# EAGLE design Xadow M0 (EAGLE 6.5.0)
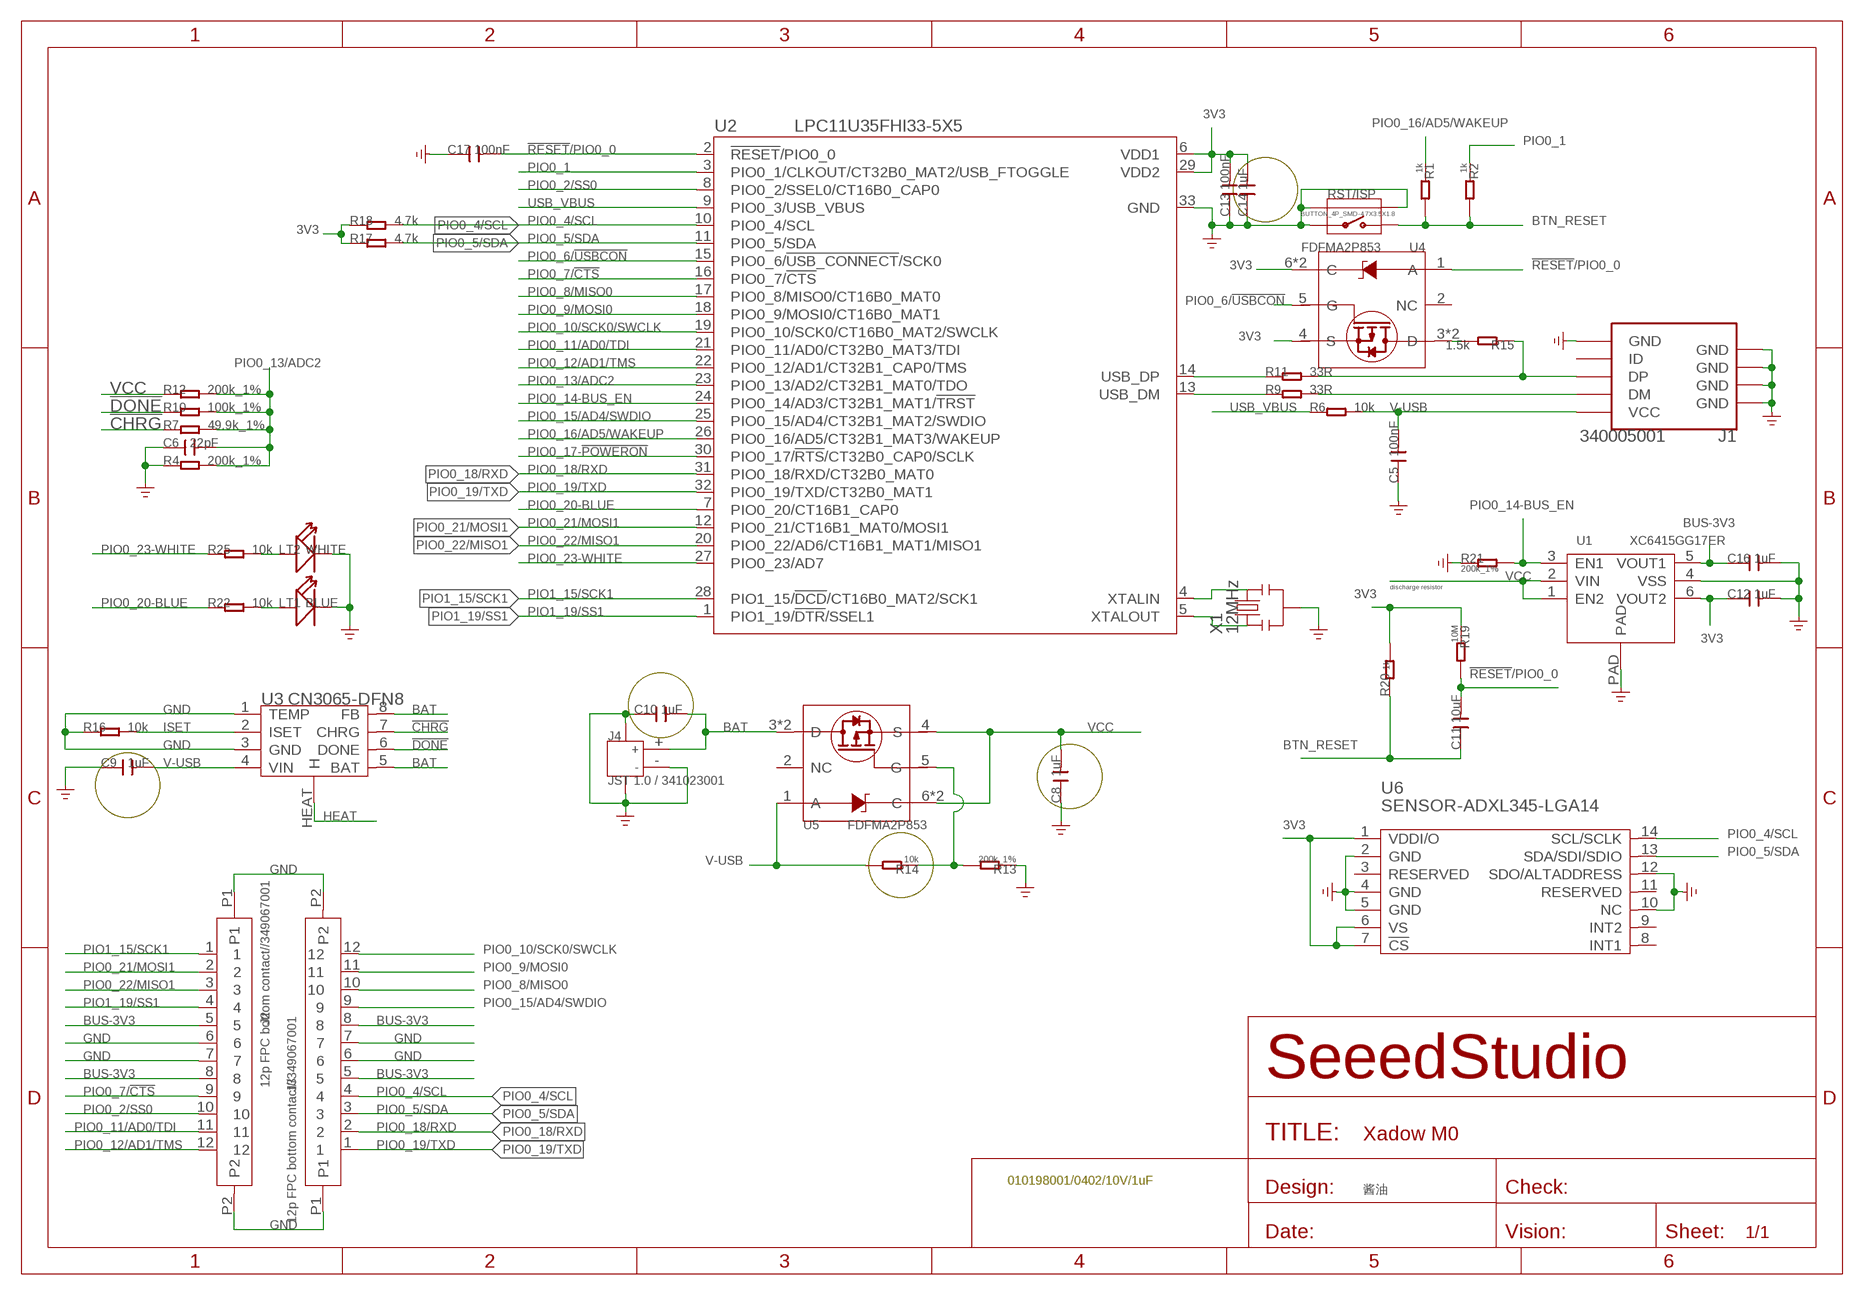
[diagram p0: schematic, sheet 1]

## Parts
C5  100nF  C-0402  [C0402]
C6  22pF  C-0402  [C0402]
C8  1uF  C-0402  [C0402]
C9  1uF  C-0402  [C0402]
C10  1uF  C-0402  [C0402]
C11  10uF  C-0402  [C0402]
C12  1uF  C-0402  [C0402]
C13  100nF  C-0402  [C0402]
C14  1uF  C-0402  [C0402]
C16  1uF  C-0402  [C0402]
C17  100nF  C-0402  [C0402]
J1  340005001  USB-MINIUSB-5P-MICRO  [MICRO-USB]
J2  12p FPC bottom contact//349067001  FPC052002-12LT-FH12-12S-0.5SH  [12P-0.5-NEW]
J3  12p FPC bottom contact//349067001  FPC052002-12LT-FH12-12S-0.5SH  [12P-0.5-NEW]
J4  JST 1.0 / 341023001  JACK-JST-2P-SMD-PW'1.0'  [JST-SMD-2P-1.0-90D]
LT1  BLUE  LED'0402'  [LED-0402]
LT2  WHITE  LED'0402'  [LED-0402]
R1  1k  R-0402  [R0402]
R2  1k  R-0402  [R0402]
R4  200k_1%  R-0402  [R0402]
R6  10k  R-0402  [R0402]
R7  49.9k_1%  R-0402  [R0402]
R9  33R  R-0402  [R0402]
R10  100k_1%  R-0402  [R0402]
R11  33R  R-0402  [R0402]
R12  200k_1%  R-0402  [R0402]
R13  200k_1%  R-0402  [R0402]
R14  10k  R-0402  [R0402]
R15  1.5k  R-0402  [R0402]
R16  10k  R-0402  [R0402]
R17  4.7k  R-0402  [R0402]
R18  4.7k  R-0402  [R0402]
R19  10M  R-0402  [R0402]
R20  1k  R-0402  [R0402]
R21  200k_1%  R-0402  [R0402]
R22  10k  R-0402  [R0402]
R25  10k  R-0402  [R0402]
RST/ISP  BUTTON_4P_SMD-4.7X3.5X1.8  [4P-SMD-4.7X3.5X1.8]
U1  XC6415GG17ER  XC6415  [USP-6C]
U2  LPC11U35FHI33-5X5  [HVQFN33]
U3  CN3065-DFN8  [DFN8]
U4  FDFMA2P853  [6P-SMD-W/-HEAT]
U5  FDFMA2P853  [6P-SMD-W/-HEAT]
U6  SENSOR-ADXL345-LGA14  [LGA14]
X1  12MHz  CRYSTAL-RESONATOR'SMD'  [3P-SMD-3.6X1.3]

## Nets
3V3: C12.1 C13.2 C14.2 R17.1 R18.1 R19.1 R20.2 U1.6(VOUT2) U2.6(VDD1) U2.29(VDD2) U4.4(S) U4.6(C) U4.P1(C) U6.1(VDDI/O) U6.6(VS) U6.7(!CS)
!CHRG: R7.1 U3.7(CHRG)
!DONE: R10.1 U3.6(DONE)
!RESET!/PIO0_0: C11.2 C17.2 R19.2 U2.2(!RESET!/PIO0_0) U4.1(A)
BAT: C10.2 J4.+ U3.5(BAT) U3.8(FB) U5.3(D) U5.P2(D)
BTN_RESET: C11.1 R1.2 R2.2 R20.1 RST/ISP.2
BUS-3V3: C16.1 J2.5 J2.8 J3.5 J3.8 U1.5(VOUT1)
GND: C5.1 C6.1 C8.1 C9.1 C10.1 C12.2 C13.1 C14.1 C16.2 C17.1 J1.5(GND) J1.S1(GND) J1.S2(GND) J1.S3(GND) J1.S4(GND) J1.S5(GND) J1.S6(GND) J2.6 J2.7 J2.P1 J2.P2 J3.6 J3.7 J3.P1 J3.P2 J4.3 J4.4 J4.- LT1.- LT2.- R4.1 R13.1 R16.1 R21.1 RST/ISP.1 RST/ISP.S1 RST/ISP.S2 U1.4(VSS) U1.PAD U2.33(GND) U3.1(TEMP) U3.3(GND) U6.2(GND) U6.4(GND) U6.5(GND) U6.10(NC) U6.12(SDO/ALTADDRESS) X1.2
HEAT: U3.HEAT(H)
ISET: R16.2 U3.2(ISET)
N$1: R11.1 U2.14(USB_DP)
N$2: R9.1 U2.13(USB_DM)
N$3: J1.2(DM) R9.2
N$4: J1.3(DP) R11.2 R15.1
N$5: LT2.+ R25.2
N$6: U2.4(XTALIN) X1.3
N$7: U2.5(XTALOUT) X1.1
N$8: R13.2 R14.1 U5.5(G)
N$9: LT1.+ R22.2
N$11: R15.2 U4.3(D) U4.P2(D)
PIO0_1: R2.1 U2.3(PIO0_1/CLKOUT/CT32B0_MAT2/USB_FTOGGLE)
PIO0_2/SS0: J2.10 U2.8(PIO0_2/SSEL0/CT16B0_CAP0)
PIO0_4/SCL: J3.4 R18.2 U2.10(PIO0_4/SCL) U6.14(SCL/SCLK)
PIO0_5/SDA: J3.3 R17.2 U2.11(PIO0_5/SDA) U6.13(SDA/SDI/SDIO)
PIO0_6/!USBCON: U2.15(PIO0_6/!USB_CONNECT!/SCK0) U4.5(G)
PIO0_7/!CTS: J2.9 U2.16(PIO0_7/!CTS!)
PIO0_8/MISO0: J3.10 U2.17(PIO0_8/MISO0/CT16B0_MAT0)
PIO0_9/MOSI0: J3.11 U2.18(PIO0_9/MOSI0/CT16B0_MAT1)
PIO0_10/SCK0/SWCLK: J3.12 U2.19(PIO0_10/SCK0/CT16B0_MAT2/SWCLK)
PIO0_11/AD0/TDI: J2.11 U2.21(PIO0_11/AD0/CT32B0_MAT3/TDI)
PIO0_12/AD1/TMS: J2.12 U2.22(PIO0_12/AD1/CT32B1_CAP0/TMS)
PIO0_13/ADC2: C6.2 R4.2 R7.2 R10.2 R12.2 U2.23(PIO0_13/AD2/CT32B1_MAT0/TDO)
PIO0_14-BUS_EN: R21.2 U1.3(EN1) U2.24(PIO0_14/AD3/CT32B1_MAT1/!TRST!)
PIO0_15/AD4/SWDIO: J3.9 U2.25(PIO0_15/AD4/CT32B1_MAT2/SWDIO)
PIO0_16/AD5/WAKEUP: R1.1 U2.26(PIO0_16/AD5/CT32B1_MAT3/WAKEUP)
PIO0_17-!POWERON: U2.30(PIO0_17/!RTS!/CT32B0_CAP0/SCLK)
PIO0_18/RXD: J3.2 U2.31(PIO0_18/RXD/CT32B0_MAT0)
PIO0_19/TXD: J3.1 U2.32(PIO0_19/TXD/CT32B0_MAT1)
PIO0_20-BLUE: R22.1 U2.7(PIO0_20/CT16B1_CAP0)
PIO0_21/MOSI1: J2.2 U2.12(PIO0_21/CT16B1_MAT0/MOSI1)
PIO0_22/MISO1: J2.3 U2.20(PIO0_22/AD6/CT16B1_MAT1/MISO1)
PIO0_23-WHITE: R25.1 U2.27(PIO0_23/AD7)
PIO1_15/SCK1: J2.1 U2.28(PIO1_15/!DCD!/CT16B0_MAT2/SCK1)
PIO1_19/SS1: J2.4 U2.1(PIO1_19/!DTR!/SSEL1)
USB_VBUS: R6.1 U2.9(PIO0_3/USB_VBUS)
V-USB: C5.2 C9.2 J1.1(VCC) R6.2 R14.2 U3.4(VIN) U5.1(A)
VCC: C8.2 R12.1 U1.1(EN2) U1.2(VIN) U5.4(S) U5.6(C) U5.P1(C)
Unconnected: J1.4(ID) U4.2(NC) U5.2(NC) U6.3(RESERVED) U6.8(INT1) U6.9(INT2) U6.11(RESERVED)

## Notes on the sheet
- discharge resistor
- 010198001/0402/10V/1uF
- 酱油

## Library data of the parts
C5 C6 C8-C14 C16 C17 = Discrete:C*: Ceramic Capacitors
J1 = Connector :USB-MINIUSB-5P
J2 J3 = template:FPC052002-12LT
J4 = Connector :JACK-JST-2P-SMD-PW
LT1 LT2 = Discrete:LED*
R1 R2 R4 R6 R7 R9-R22 R25 = Discrete:R*
RST/ISP = For_Test_Albert:BUTTON_4P_SMD: TS-1188E http://www.best-dz.com/?thread-374-2.html
U1 = template :XC6415: Dual LDO Regulator with ON/OFF Switch
U2 = For_Test_Albert:LPC11U35FHI33
U3 = IC:CN3065: USB-Compatible Lithiumt-Ion Battery Charger with Thermal Regulation http://www.consonance-elec.com/pdf/%E6%8A%80%E6%9C%AF%E8%AF%B4%E6%98%8E%E4%B9%A6/DSC-CN3065.pdf
U4 = template:FDFMA2P853: Integrated P-Channel Power Trench MOSFET and Schottky Diode
U5 = template :FDFMA2P853: Integrated P-Channel Power Trench MOSFET and Schottky Diode
U6 = Discrete:SENSOR-ADXL345: 3-Axis,+/-2g / +/-4g / +/-8g / +/-16g Digital Accelerometer http://www.analog.com/static/imported-files/data_sheets/ADXL345.pdf
X1 = Discrete:CRYSTAL-RESONATOR: Resonator Small SMD resonator. This is the itty bitty 10/20MHz resonators with built in caps. CSTCE10M0G55 and CSTCE20M0V53. Footprint has been reviewed closely but hasn't been tested yet.

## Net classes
0 default: width 0.102 mm, drill 0.203 mm, clearance 0.102 mm

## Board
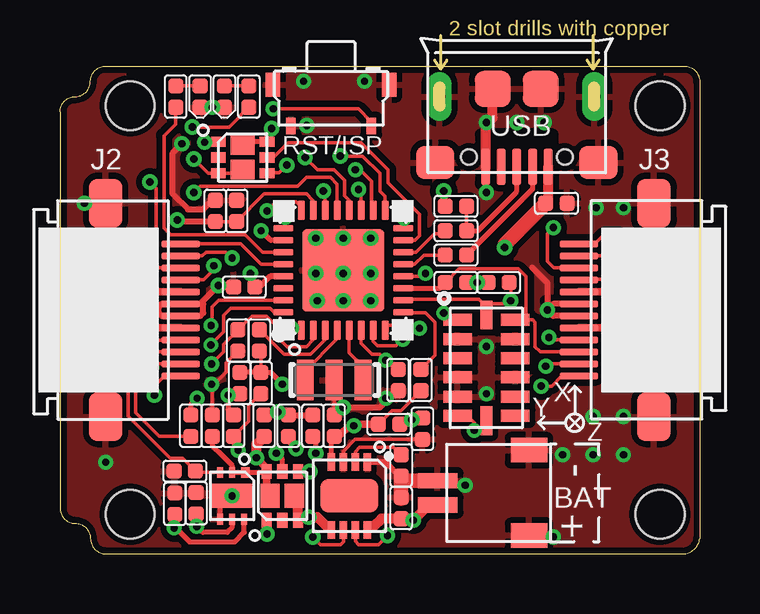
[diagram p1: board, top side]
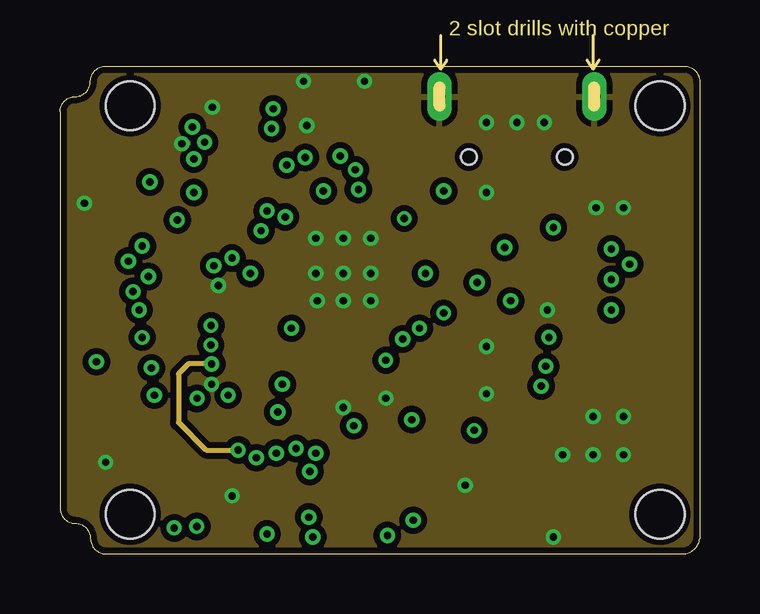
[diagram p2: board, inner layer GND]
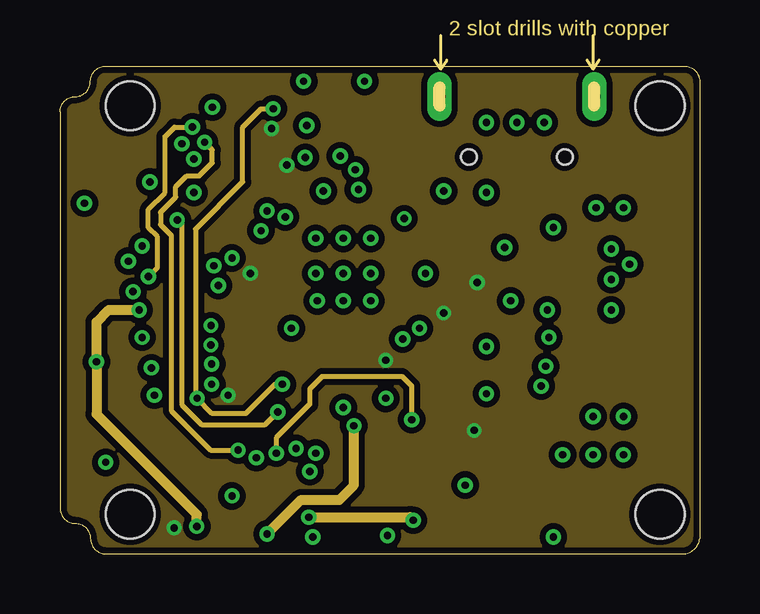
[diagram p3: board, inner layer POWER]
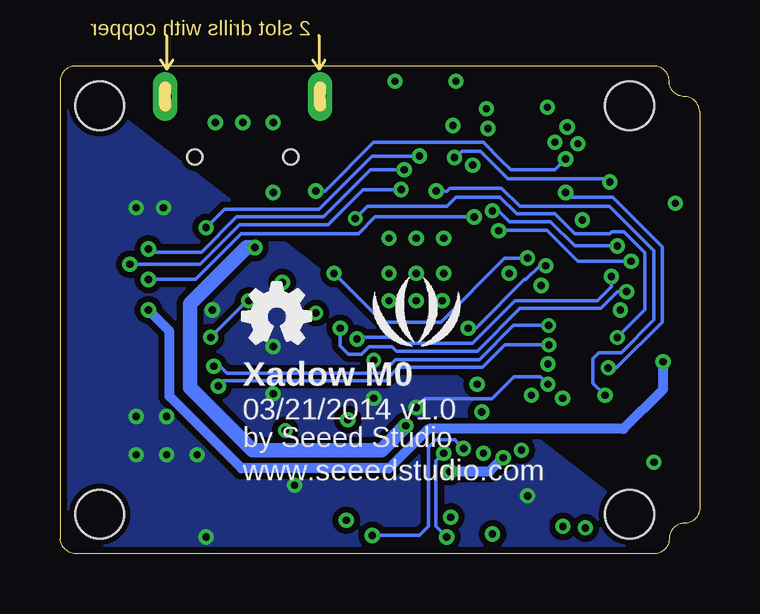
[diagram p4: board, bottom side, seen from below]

Size 26.67 x 20.32 mm. Coordinates in mm from the lower left corner, seen from the top.
Outline: 25.91,0 arc90 26.67,0.64
Outline: 26.04,20.32 arc-90 26.67,19.69
Outline: 1.27,19.69 arc-90 1.91,20.32
Outline: 0,1.91 arc90 0.64,1.27
Outline: 0,18.42 arc-90 0.64,19.05
Outline: 0.64,19.05 arc90 1.27,19.69
Outline: 0.64,1.27 arc-90 1.27,0.64
Outline: 1.27,0.64 arc90 1.91,0
Outline: 25.91,0 arc90 26.67,0.64
Outline: 26.04,20.32 arc-90 26.67,19.69
Outline: 26.67,19.69 26.67,0.64
Outline: 1.27,19.69 arc-90 1.91,20.32
Outline: 0,18.42 0,1.91
Outline: 0,1.91 arc90 0.64,1.27
Outline: 0,18.42 arc-90 0.64,19.05
Outline: 0.64,19.05 arc90 1.27,19.69
Outline: 0.64,1.27 arc-90 1.27,0.64
Outline: 1.27,0.64 arc90 1.91,0
Outline: 1.91,0 25.91,0
Outline: 1.91,20.32 26.04,20.32
Copper layers (1*2*15*16): Top 0.035mm / dielectric 0.2mm / GND 0.0175mm / dielectric 0.3mm / POWER 0.0175mm / dielectric 0.2mm / Bottom 0.035mm
Design rules "default *": minimum track width 6mil, minimum drill 12mil, track to track 6mil, track to pad 6mil, pad to pad 6mil, via to via 6mil, smd to smd 0mil, copper to edge 6mil, drill to drill 10mil, minimum pad ring 6mil, minimum via ring 6mil, stop-mask expansion 2mil, vias tented up to drill 25mil, thermal gap 10mil
Holes 2.03 mm at 2.92,1.65 25.02,18.67 25.02,1.65 2.92,18.67
tRestrict: area 20.3,9.8 to 21.5,10.5; area 3.9,9.8 to 5.1,10.5; area 9.1,6.6 to 16.3,13.8; 1 lines
bRestrict: 1 lines

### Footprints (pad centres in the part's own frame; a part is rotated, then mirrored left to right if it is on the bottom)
C0402 = smd 0.635 x 0.635: 1 -0.445,0; 2 0.445,0
MICRO-USB = smd 0.381 x 1.524: 1 -1.3,-0.25; 2 -0.65,-0.25; 3 0,-0.25; 4 0.65,-0.25; 5 1.3,-0.25 | smd 1.6 x 1.397: S1 -3.4,-0.427; S6 3.4,-0.427 | drill 0.508 pad 1.016 long: S2 -3.226,-3.175; S5 3.226,-3.175 | smd 1.5 x 1.5: S3 -1,-3.5; S4 1,-3.5 | hole 0.635: -2,-0.65; 2,-0.65
12P-0.5-NEW = smd 0.3 x 1.6: 1 -2.75,3.127; 2 -2.25,3.127; 3 -1.75,3.127; 4 -1.25,3.127; 5 -0.75,3.127; 6 -0.25,3.127; 7 0.25,3.127; 8 0.75,3.127; 9 1.25,3.127; 10 1.75,3.127; 11 2.25,3.127; 12 2.75,3.127 | smd 2.032 x 1.397: P1 -4.445,0; P2 4.445,0
JST-SMD-2P-1.0-90D = smd 1.524 x 1.016: 3 -3.429,1.778; 4 -3.429,-1.778 | smd 1.651 x 0.635: + 0.381,0.508; - 0.381,-0.508
LED-0402 = smd 0.635 x 0.635: + -0.445,0; - 0.445,0
R0402 = smd 0.635 x 0.635: 1 -0.445,0; 2 0.445,0
4P-SMD-4.7X3.5X1.8 = smd 0.4 x 0.7: 1 -1.675,-1.227; 2 1.675,-1.227 | smd 0.6 x 1: S1 -2.425,0.5; S2 2.425,0.5
USP-6C = smd 0.45 x 0.35: 1 -0.975,0.55 | smd 0.45 x 0.25: 2 -0.975,0; 3 -0.975,-0.5; 4 0.975,-0.5; 5 0.975,0; 6 0.975,0.5 | smd 1 x 1.8: PAD 0,0
HVQFN33 = smd 0.813 x 0.279: 1 -2.5,1.75; 2 -2.5,1.25; 3 -2.5,0.75; 4 -2.5,0.25; 5 -2.5,-0.25; 6 -2.5,-0.75; 7 -2.5,-1.25; 8 -2.5,-1.75; 17 2.5,-1.75; 18 2.5,-1.25; 19 2.5,-0.75; 20 2.5,-0.25; 21 2.5,0.25; 22 2.5,0.75; 23 2.5,1.25; 24 2.5,1.75 | smd 0.279 x 0.813: 9 -1.75,-2.5; 10 -1.25,-2.5; 11 -0.75,-2.5; 12 -0.25,-2.5; 13 0.25,-2.5; 14 0.75,-2.5; 15 1.25,-2.5; 16 1.75,-2.5; 25 1.75,2.5; 26 1.25,2.5; 27 0.75,2.5; 28 0.25,2.5; 29 -0.25,2.5; 30 -0.75,2.5; 31 -1.25,2.5; 32 -1.75,2.5 | smd 3.429 x 3.429: 33 0,0
DFN8 = smd 0.3 x 0.727: 1 -0.75,-1.413; 2 -0.25,-1.413; 3 0.25,-1.413; 4 0.75,-1.413; 5 0.75,1.413; 6 0.25,1.413; 7 -0.25,1.413; 8 -0.75,1.413 | smd 2.413 x 1.397: HEAT 0,0
6P-SMD-W/-HEAT = smd 0.42 x 0.62: 1 -0.65,-1.015; 2 0,-1.015; 3 0.65,-1.015; 4 0.65,1.015; 5 0,1.015; 6 -0.65,1.015 | smd 0.8 x 1: P1 -0.508,0; P2 0.5,0
LGA14 = smd 1.2 x 0.5: 1 -1.2,2; 2 -1.2,1.2; 3 -1.2,0.4; 4 -1.2,-0.4; 5 -1.2,-1.2; 6 -1.2,-2; 8 1.2,-2; 9 1.2,-1.2; 10 1.2,-0.4; 11 1.2,0.4; 12 1.2,1.2; 13 1.2,2 | smd 0.5 x 1.2: 7 0,-2.2; 14 0,2.2
3P-SMD-3.6X1.3 = smd 0.7 x 1.7: 1 -1.2,0; 2 0,0; 3 1.2,0

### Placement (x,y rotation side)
C5  20.7,14.61 180 top
C6  7.37,14.29 270 top
C8  6.35,5.34 270 top
C9  11.43,5.34 270 top
C10  14.22,1.91 270 top
C11  8.38,7.11 270 top
C12  4.79,2.09 90 top
C13  7.68,11.12 0 top
C14  14.1,7.24 90 top
C16  5.68,2.11 90 top
C17  7.42,8.89 90 top
J1  19.05,15.88 180 top
J2  1.91,10.16 270 top
J3  24.76,10.16 90 top
J4  16.13,2.54 180 top
LT1  6.86,19.05 270 top
LT2  5.84,19.05 270 top
R1  5.46,5.34 90 top
R2  8.31,8.89 270 top
R4  6.48,14.29 270 top
R6  15.05,7.24 270 top
R7  9.53,5.34 90 top
R9  16.51,12.45 0 top
R10  10.54,5.34 90 top
R11  16.51,13.46 0 top
R12  8.51,5.34 90 top
R13  15.11,5.21 90 top
R14  13.72,5.4 180 top
R15  16.51,14.48 180 top
R16  14.22,3.69 90 top
R17  16.51,11.31 180 top
R18  18.29,11.31 0 top
R19  7.24,5.34 270 top
R20  7.49,7.11 270 top
R21  5.21,3.44 0 top
R22  7.87,19.05 90 top
R25  4.83,19.05 90 top
RST/ISP  11.3,19.05 0 top
U1  7.18,2.42 270 top
U2  11.81,11.81 90 top
U3  12.06,2.42 180 top
U4  7.62,16.51 270 top
U5  9.27,2.42 0 top
U6  17.78,7.75 0 top
U$13  [OSHW_FILLX100_NOTEXT]  19.05,8.77 0 bottom
U$14  [SILK_SCREEN_150X124]  11.81,9.78 0 bottom
X1  11.43,7.24 180 top

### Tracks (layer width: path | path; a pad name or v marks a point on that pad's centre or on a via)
3V3  (via drill 0.3 pad 0.61, 0.3 pad 0.64)
  Top 0.152: U4.4 8.75,15.86 8.76,15.88 9.14,15.88 v9.46,16.2 | U2.6 12.56,8.78 13.02,8.32 13.34,8.32 v13.59,8.07 13.97,7.69 C14.2 | U6.7 17.78,5.21 17.72,5.15 v17.27,5.15 17.27,5.46 17.02,5.72 16.61,5.72 U6.6 | R18.1 v17.4,11.31 | 7.37,5.91 R19.1 | U6.1 16.29,9.75 v16,10.04
  Top 0.203: C12.1 4.79,1.12 5.41,0.5 7.29,0.5 7.68,0.89 U1.6 | v8.83,17.72 8.63,17.53 U4.6 7.76,17.16 U4.P1 | R20.2 7.07,6.67 v7.01,6.61 7.01,6.01 R19.1
  Top 0.254: v7.94,11.69 7.94,11.31 C13.2 8.19,11.05 8.26,11.05 8.77,11.56 U2.29
  Top 0.305: C12.1 4.79,1.11 v4.76,1.08
  Top 0.406: R17.1 v17.4,11.31
  pour POWER (isolate 0.254): 27.3,20.32 -3.17,20.32 -3.17,-0.63 27.3,-0.63
!CHRG  (via drill 0.3 pad 0.64)
  Top 0.152: U3.7 12.31,0.51 12.45,0.38 13.27,0.38 v13.65,0.76
  Top 0.203: 9.53,4.83 R7.1 9.53,4.7 v9.84,4.38
  Bottom 0.152: v13.65,0.76 11.68,0.76 11.3,1.15 11.3,4.44 11,4.74 10.2,4.74 10.08,4.62 v9.84,4.38
!DONE  (via drill 0.3 pad 0.64)
  Top 0.152: U3.6 11.81,0.51 11.69,0.38 10.86,0.38 v10.54,0.7
  Top 0.203: v10.67,4.19 10.67,4.76 R10.1
  Bottom 0.152: v10.67,4.19 10.98,3.88 10.98,1.15 v10.54,0.7
!RESET!/PIO0_0  (via drill 0.3 pad 0.64)
  Top 0.152: U2.2 10.56,8.91 10.29,8.64 9.47,8.64 9.02,9.1 9.02,9.5 8.61,9.91 8,9.91 7.6,9.5 7.58,9.5 C17.2 6.83,8.74 6.83,8.42 v6.33,7.91 | U4.1 6.05,17.16 v6.03,17.15 | C11.2 7.87,6.16 7.87,5.53 R19.2 7.24,4.51 v7.43,4.32
  GND 0.203: v7.43,4.32 6.1,4.32 4.94,5.47 4.94,7.5 5.36,7.91 v6.33,7.91
  POWER 0.203: v7.43,4.32 6.28,4.32 4.64,5.97 4.64,13.27 4.19,13.72 4.19,14.23 4.83,14.86 4.83,15.29 5.28,15.75 5.81,15.75 6.35,16.29 6.35,16.83 v6.03,17.15
BAT  (via drill 0.3 pad 0.64)
  Top 0.254: 12.95,1.15 12.95,1.14 U3.8
  Top 0.305: U3.8 | 11.18,1.08 11.23,1.08 U3.5
  Top 0.406: U5.3 9.92,1.53 | 9.92,1.53 9.92,2.27 U5.P2 | J4.+ 15.37,2.03 v14.73,1.4 14.29,1.4 C10.2 13.4,1.46 13.08,1.15 12.95,1.15 | 9.92,1.53 v10.38,1.53 10.73,1.53 11.18,1.08
  POWER 0.406: v10.38,1.53 14.6,1.53 v14.73,1.4
BTN_RESET  (via drill 0.3 pad 0.64)
  Top 0.152: 12.95,17.8 RST/ISP.2 12.98,18.01 12.45,18.54 v8.89,18.54 | C11.1 8.38,8.37 R2.2
  Top 0.203: R20.1 C11.1 8.78,7.56 v9.27,7.06 | R1.2 5.46,6.23 v5.71,6.48
  POWER 0.203: v8.89,18.54 8.38,18.54 7.62,17.78 7.62,15.5 5.65,13.53 5.65,6.54 v5.71,6.48 6.35,5.84 7.75,5.84 8.97,7.06 v9.27,7.06
BUS-3V3  (via drill 0.3 pad 0.64)
  Top 0.203: U1.5 7.18,1.09 6.98,0.9 5.95,0.9 v5.7,1.15 5.7,1.6 | 5.7,1.6 5.7,1.64 C16.1 | 5.7,1.6 5.65,1.65 | 21.65,10.92 J3.8
  Top 0.254: 5.02,9.4 J2.8
  Top 0.305: J2.8 4.04,9.41 4.04,9.42 v3.3,10.16 4.04,10.91 J2.5 | J3.5 22.64,9.41 22.99,9.76 v22.99,10.16 22.99,10.54 22.62,10.91 J3.8
  POWER 0.406: v3.3,10.16 2.03,10.16 1.52,9.65 v1.52,8 1.52,5.82 5.7,1.64 v5.7,1.15
  Bottom 0.406: v22.99,10.16 22.1,9.27 22.1,6.56 19.1,3.56 12.95,3.56 11.3,5.21 3.17,5.21 1.52,6.86 v1.52,8
GND  (via drill 0.3 pad 0.64)
  Top 0.152: LT2.- v6.35,18.61 LT1.- | U3.3 11.81,4.27 12.31,4.76 R13.1 | C17.1 6.92,7.95 6.92,7.56 6.43,7.06 v6.33,7.06 6.35,7.04 C8.1 | X1.2 11.43,6.1 v11.81,6.1
  Top 0.203: U1.4 6.68,2.3 6.79,2.42 U1.PAD
  Top 0.254: 5.84,10.41 J2.6 4.24,10.42 4.09,10.26 4.09,10.07 4.24,9.91 J2.7 5.85,9.91 5.97,10.04 5.97,10.42 | 5.84,10.41 5.97,10.54 | C13.1 6.54,11.11 | U3.1 13.57,3.83 14.22,3.18 14.16,3.18 R16.1 | 5.97,10.42 5.97,10.54 | 5.97,10.54 6.54,11.11 | 6.54,11.11 v6.6,11.18 | 5.84,10.41 5.96,10.41 5.97,10.42 | 21.47,10.41 J3.7 20.57,10.41 v20.32,10.16 | 21.72,9.91 21.71,9.91 J3.6 20.57,9.91 v20.32,10.16 | v13.59,6.48 13.59,6.35 13.34,6.1 v11.81,6.1 11.56,6.1 | 19.68,11.94 20.32,11.31 v20.32,10.16 | R4.1 6.35,14.73 5.97,14.35 5.33,14.35 4.7,14.99 4.7,16.7 v5.08,17.08
  Top 0.305: J2.P1 v1.02,14.61
  Top 0.406: 17.75,17.88 18.03,18.16 18.03,19.36 J1.S4 | 11.56,6.1 11.56,5.91 C9.1 | J1.5 17.75,18.01 17.78,18.04
  Top 0.61: J4.- 14.22,3.05 | 14.22,3.05 14.22,3.18 R16.1 | 14.22,3.05 14.22,2.29 | U2.33 11.81,11.88
  Bottom 0.152: v6.33,7.06 6.63,7.37 7.75,7.37 8.66,6.45 11.46,6.45 v11.81,6.1
  other vias: 23.49,5.72 10.73,10.54 11.81,10.54 12.95,10.54 10.29,17.85 10.16,19.69 20.95,4.13 16.89,2.86 20.57,0.7 17.78,17.97 19.05,17.97 20.19,17.97 10.67,13.15 11.81,13.15 12.95,13.15 11.81,11.69 10.67,11.69 12.95,11.69 7.18,2.42 1.91,3.81 17.78,8.64 17.78,15.05 22.35,14.42 12.7,19.69 17.78,6.67 23.49,14.42 22.22,5.72 22.22,4.13 23.49,4.13
  pour GND (isolate 0.254): 27.3,20.32 -2.54,20.32 -2.54,-0.63 27.3,-0.63
  pour Bottom (isolate 0.254, rank 4): 27.3,20.7 27.3,-0.63 -0.25,-0.63
  pour Top (isolate 0.254, rank 4): -0.25,20.7 27.3,20.7 27.3,-0.63 -0.25,-0.63
ISET
  Top 0.152: U3.2 12.31,4.26 12.49,4.44 13.91,4.44 R16.2 | R16.2 14.29,4.13 | 14.1,4.26 R16.2
N$1
  Top 0.152: U2.14 14.85,12.56 15.62,13.34 15.94,13.34 R11.1
N$2
  Top 0.152: U2.13 14.79,12.06 15.18,12.45 R9.1
N$3
  Top 0.203: J1.2 19.7,15.19 18.61,14.1 17.53,13.02 R9.2
N$4
  Top 0.152: R15.1 R11.2
  Top 0.203: R11.2 17.42,13.46 19.05,15.09 J1.3
N$5
  Top 0.152: R25.2 LT2.+
N$6
  Top 0.152: U2.4 11.56,8.96 10.23,7.63 X1.3
N$7
  Top 0.152: U2.5 12.06,8.39 12.64,7.81 12.64,7.25 X1.1
N$8  (via drill 0.3 pad 0.64)
  Top 0.203: U5.5 9.27,3.94 v9.02,4.19
  Top 0.254: R14.1 14.48,5.4 v14.67,5.59 14.73,5.65 R13.2
  POWER 0.203: v14.67,5.59 14.67,6.98 14.26,7.39 10.95,7.39 10.41,6.86 10.41,6.23 9.02,4.83 v9.02,4.19
N$9
  Top 0.152: LT1.+ R22.2
N$11  (via drill 0.3 pad 0.64)
  Top 0.152: U4.3 7.47,15.86 U4.P2 | 6.49,15.75 U4.3 | v16,15.12 16,14.54 R15.2 | U4.3 6.17,15.86 v5.59,16.45
  Bottom 0.152: v16,15.12 15.62,15.12 13.6,17.14 9.02,17.14 8.26,16.39 7.87,16 6.03,16 v5.59,16.45
PIO0_1
  Top 0.152: U2.3 11.06,8.93 10.45,8.32 9.34,8.32 9.27,8.38 8.51,9.15 8.5,9.15 R2.1
PIO0_2/SS0  (via drill 0.3 pad 0.64)
  Top 0.152: U2.8 13.56,9.5 13.59,9.53 14.86,9.53 v14.99,9.4 | J2.10 3.22,8.41 2.71,8.93 2.71,10.59 v3.05,10.92
  Bottom 0.152: v14.99,9.4 14.99,8.66 14.64,8.32 14.1,8.32 13.78,8.64 12.83,8.64 12.64,8.45 9.27,8.45 7.49,10.23 4.13,10.23 3.43,10.92 v3.05,10.92
PIO0_4/SCL  (via drill 0.3 pad 0.64)
  Top 0.152: U2.10 14.62,10.56 14.67,10.61 17.46,10.61 17.78,10.29 | U6.14 17.78,10.29 | J3.4 20.49,8.91 v20.38,9.02 | 17.78,10.29 17.91,10.42 18.67,10.42 v18.8,10.54 18.8,11.24 R18.2
  Bottom 0.152: v20.38,9.02 18.99,10.42 18.86,10.54 v18.8,10.54
PIO0_5/SDA
  Top 0.152: 16.07,11.24 R17.2 16.64,11.88 19.11,11.88 19.43,11.56 19.43,9.78 | J3.3 20.04,8.41 19.81,8.64 19.81,9.65 19.72,9.75 19.46,9.75 | 19.43,9.78 19.43,9.75 | U6.13 19.46,9.75 | 19.46,9.75 19.43,9.78
  Top 0.203: U2.11 15.82,11.06 R17.2
PIO0_6/!USBCON
  Top 0.152: U2.15 14.79,13.06 14.99,13.26 14.99,14.16 13.69,15.46 13.69,16.01 12.56,17.13 9.51,17.13 8.89,16.51 U4.5
PIO0_7/!CTS  (via drill 0.3 pad 0.61)
  Top 0.152: J2.9 5.01,8.89 3.56,8.89 v3.43,9.02 | U2.16 14.31,13.93 v14.35,13.97
  Bottom 0.152: v14.35,13.97 13.84,14.48 10.54,14.48 10.15,14.87 8.32,14.87 7.62,14.16 6.03,14.16 5.21,13.34 3.75,13.34 3.66,13.42 3.15,13.42 2.29,12.55 2.29,10.16 v3.43,9.02
PIO0_8/MISO0  (via drill 0.3 pad 0.64)
  Top 0.152: v11.68,16.58 12.62,16.58 13.34,15.86 13.34,15.12 13.56,14.89 U2.17 | 21.67,11.94 J3.10 20.6,11.91 20.32,12.19 20.32,13.34 v20.57,13.59
  Bottom 0.152: v11.68,16.58 13.65,16.58 15.88,14.35 19.81,14.35 v20.57,13.59
PIO0_9/MOSI0  (via drill 0.3 pad 0.64)
  Top 0.152: v12.32,16 12.51,16 13,15.52 13,14.69 13.08,14.61 13.08,14.33 U2.18 | J3.11 22.7,12.41 v22.99,12.7
  Bottom 0.152: v12.32,16 13.72,16 15.69,14.04 19.3,14.04 20.76,12.58 22.86,12.58 v22.99,12.7
PIO0_10/SCK0/SWCLK  (via drill 0.3 pad 0.64)
  Top 0.152: U2.19 12.56,15.06 v12.45,15.18 | v23.75,12.07 23.75,12.87 23.31,13.31 22.7,13.31 22.31,12.91 J3.12
  Bottom 0.152: v23.75,12.07 20.83,12.07 19.18,13.72 15.49,13.72 14.03,15.18 v12.45,15.18
PIO0_11/AD0/TDI  (via drill 0.3 pad 0.64)
  Top 0.152: U2.21 11.56,15.4 11.27,15.69 10.29,15.69 9.91,15.31 5.84,15.31 v5.59,15.05 | J2.11 3.97,7.91 v3.81,7.75
  Bottom 0.152: v3.81,7.75 3.47,7.75 1.56,9.66 1.56,12.8 3.62,14.86 5.4,14.86 v5.59,15.05
PIO0_12/AD1/TMS  (via drill 0.3 pad 0.64)
  Top 0.152: U2.22 11.06,15.04 v10.98,15.12 | v3.94,6.61 3.94,6.99 4.36,7.41 J2.12
  Bottom 0.152: v10.98,15.12 10.54,15.12 10.41,15.24 8.26,15.24 7.49,14.48 3.76,14.48 1.91,12.63 1.91,9.75 3.27,8.38 4.19,8.38 4.45,8.13 4.45,7.11 v3.94,6.61
PIO0_13/ADC2  (via drill 0.3 pad 0.64)
  Top 0.152: R4.2 C6.2 8.52,14.99 10.28,14.99 10.54,14.73 10.54,14.5 10.56,14.48 | U2.23 10.56,14.48 | 10.56,14.48 10.56,14.59
  Top 0.203: 9.5,5.76 R7.2 9.46,5.78 | R12.2 8.65,5.78
  Top 0.254: R10.2 R7.2 9.21,5.78 v9.08,5.91 8.64,5.91 R12.2 | R4.2 4.95,13.85 v4.89,13.91
  POWER 0.203: v4.89,13.91 5.08,13.72 5.08,6.22 5.91,5.38 8.56,5.38 v9.08,5.91
PIO0_14-BUS_EN  (via drill 0.3 pad 0.64)
  Top 0.152: U2.24 10.06,14.45 9.85,14.67 9.01,14.67 8.95,14.6 v8.64,14.29 | v3.43,12.83 2.54,12.83 2.07,12.36 2.07,8.48 2.84,7.7 2.84,5.74 4.6,3.99 5.11,3.99 R21.2 5.71,3.39 U1.3
  Bottom 0.152: v3.43,12.83 5.21,12.83 6.22,13.85 7.94,13.85 8.38,14.29 v8.64,14.29
PIO0_15/AD4/SWDIO  (via drill 0.3 pad 0.64)
  Top 0.152: v9.4,14.04 9.4,13.65 U2.25 | v22.99,11.43 21.66,11.43 J3.9
  Bottom 0.152: v22.99,11.43 21.02,11.43 19.11,13.34 14.22,13.34 13.53,14.04 v9.4,14.04
PIO0_16/AD5/WAKEUP  (via drill 0.3 pad 0.64)
  Top 0.152: v2.86,12.19 2.38,11.71 2.38,8.68 3.15,7.9 3.15,5.87 4.13,4.89 R1.1
  Top 0.203: U2.26 8.78,13.06 v8.38,13.46
  Bottom 0.152: v8.38,13.46 8.36,13.49 6.37,13.49 5.08,12.19 v2.86,12.19
PIO0_18/RXD  (via drill 0.3 pad 0.61, 0.3 pad 0.64)
  Top 0.152: 20.32,7.88 v20.26,7.81 20.36,7.91 J3.2 | U2.31 6.62,10.56 6.35,10.29 6.35,9.57 v6.3,9.51
  Bottom 0.152: v20.26,7.81 20,7.81 19.71,7.52 13.26,7.52 12.69,8.09 9.19,8.09 7.76,9.51 v6.3,9.51
PIO0_19/TXD  (via drill 0.3 pad 0.61, 0.3 pad 0.64)
  Top 0.152: J3.1 20.93,7.41 20.51,6.99 v20.07,6.99 | U2.32 8.93,10.06 8.76,10.23 7.11,10.23 6.83,9.95 6.83,9.25 v6.29,8.7
  Bottom 0.152: v20.07,6.99 19.84,7.22 13.11,7.22 12.55,7.77 9.06,7.77 8.13,8.7 v6.29,8.7
PIO0_20-BLUE  (via drill 0.3 pad 0.64)
  Top 0.152: U2.7 13.06,8.85 13.24,8.67 14,8.67 v14.29,8.96 | R22.1 7.05,17.78 v5.53,17.78
  POWER 0.203: v5.53,17.78 4.78,17.78 4.38,17.39 4.38,15.05 3.68,14.35 3.68,13.59 4.06,13.21 4.06,11.94 v3.68,11.56
  Bottom 0.152: v3.68,11.56 3.68,11.13 4.27,10.54 7.7,10.54 9.47,8.77 12.45,8.77 12.7,9.02 14.22,9.02 v14.29,8.96
PIO0_21/MOSI1  (via drill 0.3 pad 0.64)
  Top 0.152: J2.2 5.93,12.41 6.1,12.58 6.92,12.58 v7.18,12.32 | U2.12 15.12,11.56 v15.24,11.69
  Bottom 0.152: v7.18,12.32 v7.18,12.31 8.13,12.31 10.79,9.65 13.21,9.65 13.34,9.78 v15.24,11.69
PIO0_22/MISO1  (via drill 0.3 pad 0.64)
  Top 0.152: U2.20 12.06,14.74 11.87,14.93 11.87,15.56 11.43,16 10.73,16 v10.22,16.51 | 5,11.94 J2.3 4.14,11.91 4,12.05 4,15.24 v3.75,15.5
  Bottom 0.152: 3.87,15.62 8,15.62 | 8,15.62 9.14,16.77 9.91,16.77 10.16,16.51 v10.22,16.51 | 3.87,15.62 v3.75,15.5 | 3.87,15.62 8,15.62
PIO0_23-WHITE
  Top 0.152: U2.27 8.46,12.56 7.73,13.29 4.62,13.29 4.34,13.57 4.34,17.42 4.83,17.91 R25.1
PIO1_15/SCK1
  Top 0.152: U2.28 8.39,12.06 7.54,12.91 J2.1
PIO1_19/SS1  (via drill 0.3 pad 0.64)
  Top 0.152: v9.65,9.4 9.97,9.4 U2.1 | J2.4 5.99,11.41 6.41,11.83 v6.41,12
  Bottom 0.152: v9.65,9.4 9.34,9.4 7.3,11.43 7.24,11.43 6.67,12 v6.41,12
USB_VBUS
  Top 0.152: U2.9 14.34,10.04 15.24,10.04 15.63,9.64 15.63,8.27 R6.1
V-USB  (via drill 0.3 pad 0.64)
  Top 0.152: R14.2 13.84,5.97 14.22,5.97 R6.2
  Top 0.203: U5.1 8.62,0.84 v8.64,0.83 | U3.4 11.31,4.78 C9.2
  Top 0.305: C9.2 11.49,4.96 11.68,4.96 12.06,5.34 v12.26,5.34 12.32,5.4 R14.2
  Top 0.406: J1.1 20.35,14.7 C5.2
  Top 0.61: v18.54,12.77 18.54,12.89 C5.2
  POWER 0.406: v8.64,0.83 10.06,2.25 11.65,2.25 12.26,2.86 v12.26,5.34
  Bottom 0.61: v18.54,12.77 18.89,12.77 21.24,10.41 21.24,6.92 18.64,4.32 13.27,4.32 v12.26,5.34
VCC  (via drill 0.3 pad 0.64)
  Top 0.152: U5.4 v10.41,3.43
  Top 0.203: 8.64,3.43 U5.6 8.58,3.39 U1.1 U1.2 7.18,3.69 6.61,4.25 6.48,4.38 6.35,4.51 C8.2
  Top 0.305: v8.19,4 8.62,3.57 U5.6 8.62,2.56 U5.P1
  Top 0.406: v8.19,4 8.19,4.57 R12.1
  Bottom 0.406: v10.41,3.43 8.76,3.43 v8.19,4

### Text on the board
tPlace: USB | X | Y | Z | - | BAT | +
bPlace: Xadow M0 | 03/21/2014 v1.0 | by Seeed Studio | www.seeedstudio.com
